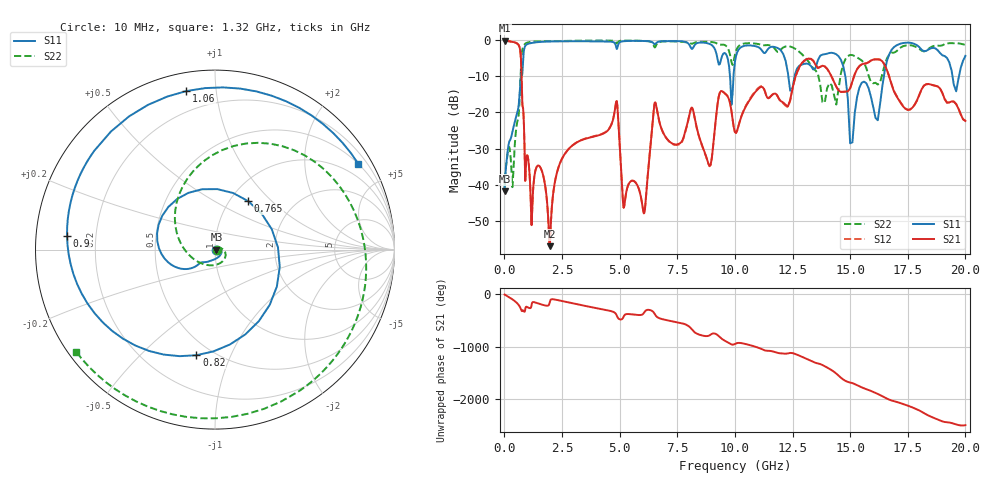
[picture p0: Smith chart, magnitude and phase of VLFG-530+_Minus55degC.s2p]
! Mini-Circuits
! S2P DATA File Format
! Type: LOW PASS FILTER
! Model: VLFG-530+
! All S Parameters are in dB deg format
! TEST CONDITIONS: INPUT POWER = 0 dBm @ Temperature = -55 deg C
# MHz S dB R 50
!Frequency  S11 dB  S11 DEG  S21 dB  S21 DEG  S12 dB  S12 DEG  S22 dB  S22 DEG
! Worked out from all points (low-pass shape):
!   652 points, 10 MHz to 20 GHz, reference 50 ohm
!   highest |S21| = -0.08 dB at 10 MHz (marker M1); lowest = -57.0 dB at 1.96 GHz (marker M2)
!   |S21| within 3 dB of the highest: start of sweep to 690.8 MHz
!   lowest |S11| = -41.8 dB at 10 MHz (marker M3), VSWR 1.02, Z = 50.8 + j0.0555 ohm
!   |S11| at or under -10 dB: start of sweep to 711.5 MHz; 14.79 GHz to 16.46 GHz (1.674 GHz wide, 10.7 % of centre); 19.44 GHz to 19.72 GHz (279.9 MHz wide, 1.43 % of centre)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
!   |S22| runs from -41.4 to -0.1 dB; largest |S21 - S12| = 0.012
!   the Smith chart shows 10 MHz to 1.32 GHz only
!   S11 on the Smith chart (normalised r, x): 10 MHz: 1.02, +0.00; 765 MHz: 1.21, +0.73; 820 MHz: 0.41, -0.75; 900 MHz: 0.09, +0.04; 1.06 GHz: 0.09, +0.83; 1.32 GHz: 0.50, +3.56
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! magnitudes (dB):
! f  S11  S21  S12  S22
! 10 MHz  -41.8  -0.1  -0.1  -41.4
! 200 MHz  -28.4  -0.3  -0.3  -29.6
! 355 MHz  -25.1  -0.4  -0.4  -40.4
! 765 MHz  -9.7  -14.5  -14.5  -3.2
! 820 MHz  -4.5  -19.5  -19.5  -1.7
! 900 MHz  -1.6  -38.2  -38.2  -1.0
! 1.06 GHz  -0.9  -34.4  -34.4  -0.5
! 1.32 GHz  -0.6  -36.9  -36.9  -0.4
! 1.96 GHz  -0.3  -57.0  -56.9  -0.2
! 2.38 GHz  -0.3  -34.6  -34.6  -0.2
! 3.35 GHz  -0.3  -27.7  -27.6  -0.1
! 4.85 GHz  -1.9  -17.0  -16.9  -0.7
! 5.175 GHz  -0.3  -46.4  -46.4  -0.1
! 6.05 GHz  -0.2  -47.9  -47.9  -0.2
! 6.675 GHz  -0.4  -21.2  -21.2  -0.6
! 8.85 GHz  -0.9  -34.1  -34.2  -0.4
! 9.45 GHz  -4.3  -14.1  -14.1  -1.2
! 10.05 GHz  -4.4  -25.7  -25.7  -2.9
! 13.4 GHz  -8.1  -5.7  -5.7  -7.8
! 15.2 GHz  -20.1  -9.4  -9.4  -4.4
! 16.7 GHz  -3.8  -10.2  -10.1  -3.9
! 20 GHz  -4.3  -22.4  -22.3  -1.3
